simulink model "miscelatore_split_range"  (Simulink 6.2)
settings: Solver=ode15s  StartTime=0.0  StopTime=5000  RelTol=1e-3
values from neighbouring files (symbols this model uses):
  A = pi    (= 3.14159265359)    [dati_miscelatore.m]
  c = 4200    [dati_miscelatore.m]
  k = 0.36    [dati_miscelatore.m]
  R = ((c*w1+c*w2+k*A)*T-c*w1*T1-c*w2*T2-k*A*Ta)/(i^2)    (= 7560)    [dati_miscelatore.m]
  rho = 1000    [dati_miscelatore.m]
  T1 = 273+50    (= 323)    [dati_miscelatore.m]
  T2 = 273+10    (= 283)    [dati_miscelatore.m]
  Ta = 273+20    (= 293)    [dati_miscelatore.m]
undefined symbols (not defined in the file or in its folder): miscelatore

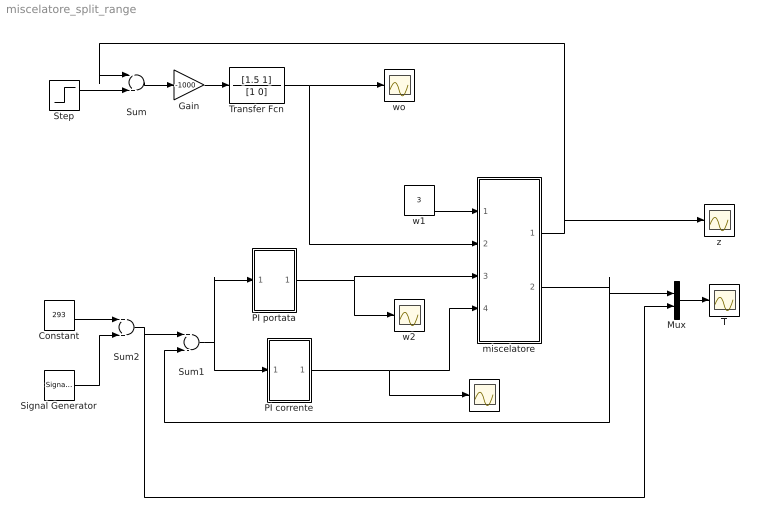
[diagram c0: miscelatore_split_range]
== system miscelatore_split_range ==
  Constant : Constant  Value=293
  Gain : Gain  Gain=-1000
  Mux : Mux  Inputs=2
  PI corrente : Subsystem
  PI portata : Subsystem
  Signal Generator : SignalGenerator  WaveForm=square  Amplitude=5  Frequency=.0005
  Step : Step  Time=0  Before=1  SampleTime=0
  Sum : Sum  Inputs=-+
  Sum1 : Sum  Inputs=+-
  Sum2 : Sum
  T : Scope
  Transfer Fcn : TransferFcn  Numerator=[1.5 1]  Denominator=[1 0]
  i : Scope
  miscelatore : Subsystem
  w1 : Constant  Value=3
  w2 : Scope
  wo : Scope
  z : Scope
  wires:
  w1/1 -> miscelatore/1(In1)
  miscelatore/1(Out1) -> Sum/1, z/1
  miscelatore/2(Out2) -> Sum1/2, Mux/1
  Step/1 -> Sum/2
  Sum1/1 -> PI portata/1(In1), PI corrente/1(In1)
  Sum2/1 -> Sum1/1, Mux/2
  Constant/1 -> Sum2/1
  Signal Generator/1 -> Sum2/2
  Gain/1 -> Transfer Fcn/1
  Sum/1 -> Gain/1
  PI corrente/1(Out1) -> miscelatore/4(In4), i/1
  PI portata/1(Out1) -> miscelatore/3(In3), w2/1
  Transfer Fcn/1 -> miscelatore/2(In2), wo/1
  Mux/1 -> T/1

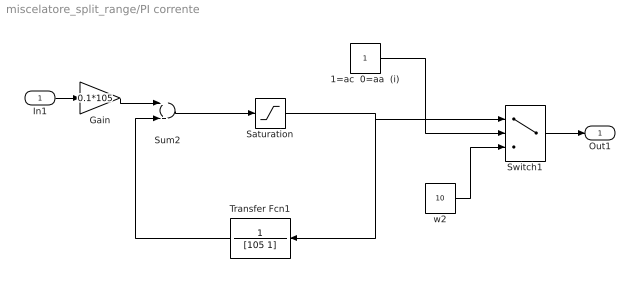
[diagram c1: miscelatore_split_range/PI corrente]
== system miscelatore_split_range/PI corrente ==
  In1 : Inport  Port=1  LatchInput=off
  1=ac  0=aa  (i) : Constant
  Gain : Gain  Gain=0.1*105
  Saturation : Saturate  UpperLimit=20  LowerLimit=0
  Sum2 : Sum
  Switch1 : Switch  Criteria=u2 > Threshold  Threshold=0.5
  Transfer Fcn1 : TransferFcn  Orientation=left  Numerator=1  Denominator=[105 1]
  w2 : Constant  Value=10
  Out1 : Outport
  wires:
  Gain/1 -> Sum2/1
  Transfer Fcn1/1 -> Sum2/2
  In1/1 -> Gain/1
  Saturation/1 -> Transfer Fcn1/1, Switch1/1
  Sum2/1 -> Saturation/1
  1=ac  0=aa  (i)/1 -> Switch1/2
  w2/1 -> Switch1/3
  Switch1/1 -> Out1/1

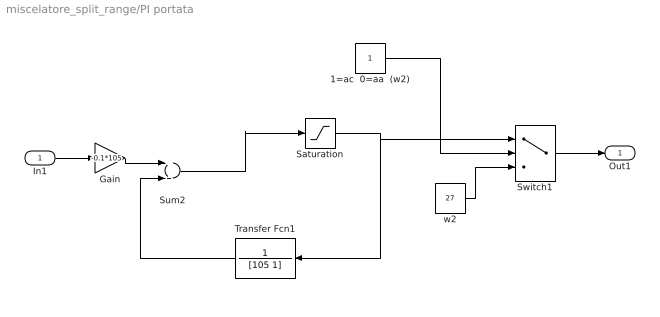
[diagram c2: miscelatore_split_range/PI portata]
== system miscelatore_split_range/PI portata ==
  In1 : Inport  Port=1  LatchInput=off
  1=ac  0=aa  (w2) : Constant
  Gain : Gain  Gain=-0.1*105
  Saturation : Saturate  UpperLimit=40  LowerLimit=15
  Sum2 : Sum
  Switch1 : Switch  Criteria=u2 > Threshold  Threshold=0.5
  Transfer Fcn1 : TransferFcn  Orientation=left  Numerator=1  Denominator=[105 1]
  w2 : Constant  Value=27
  Out1 : Outport
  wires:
  Gain/1 -> Sum2/1
  Transfer Fcn1/1 -> Sum2/2
  In1/1 -> Gain/1
  Saturation/1 -> Transfer Fcn1/1, Switch1/1
  Sum2/1 -> Saturation/1
  Switch1/1 -> Out1/1
  1=ac  0=aa  (w2)/1 -> Switch1/2
  w2/1 -> Switch1/3

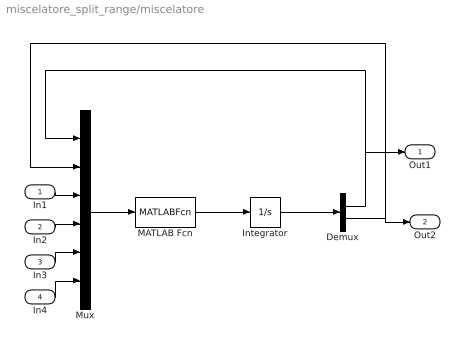
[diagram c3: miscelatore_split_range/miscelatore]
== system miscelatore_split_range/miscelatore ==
  In1 : Inport  Port=1  LatchInput=off
  In2 : Inport  Port=2  LatchInput=off
  In3 : Inport  Port=3  LatchInput=off
  In4 : Inport  Port=4  LatchInput=off
  Demux : Demux  Outputs=2
  Integrator : Integrator  InitialCondition=[1 273+20]
  MATLAB Fcn : MATLABFcn  MATLABFcn=miscelatore(u,rho,A,c,T1,T2,Ta,k,R)  OutputDimensions=2
  Mux : Mux  Inputs=6
  Out1 : Outport
  Out2 : Outport  Port=2
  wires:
  Mux/1 -> MATLAB Fcn/1
  Demux/1 -> Mux/1, Out1/1
  Demux/2 -> Mux/2, Out2/1
  MATLAB Fcn/1 -> Integrator/1
  Integrator/1 -> Demux/1
  In1/1 -> Mux/3
  In2/1 -> Mux/4
  In3/1 -> Mux/5
  In4/1 -> Mux/6
